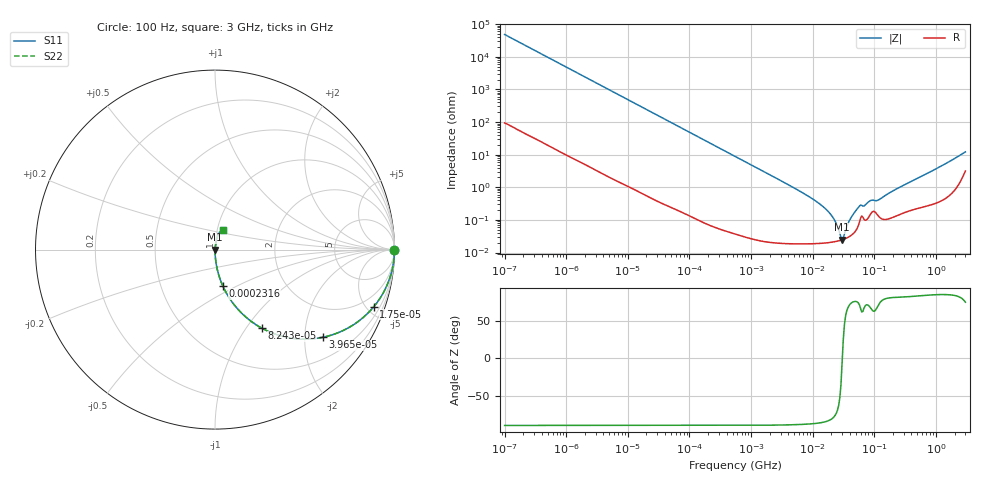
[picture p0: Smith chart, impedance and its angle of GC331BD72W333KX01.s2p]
!Murata Part Number: GC331BD72W333KX01
!These Parameters are Measured in Series Mode Connection
!Data Generated on Jun 10, 2025
!  o--ll--o
!Port1  Port2
!  o------o
!Operation Temp=25[degC], DC Bias Voltage=0[V]
!Freq. Start=100[Hz] Stop=3[GHz] 401[Steps]
# Hz S RI R 50
!Freq.(Hz) S11(Real) S11(Imag) S21(Real) S21(Imag) S12(Real) S12(Imag) S22(Real) S22(Imag)
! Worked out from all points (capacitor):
!   401 points, 100 Hz to 3 GHz, reference 50 ohm
!   read as one part in series: C = 32.9 nF near 109 Hz
!   lowest |Z| = 24.7 mohm at 29.99 MHz (marker M1)
!   series resonance near 30.23 MHz, so ESL is about 840 pH
!   S11 on the Smith chart (normalised r, x): 100 Hz: open; 17.5 kHz: 1.01, -5.56; 39.66 kHz: 1.01, -2.46; 82.43 kHz: 1.00, -1.18; 231.6 kHz: 1.00, -0.42; 3 GHz: 1.06, +0.24
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100  1 -0.00207  8.3e-06 0.00207  8.3e-06 0.00207  1 -0.00207
1788  0.9986 -0.0368  0.00143 0.0368  0.00143 0.0368  0.9986 -0.0368
6230  0.9836 -0.126  0.0164 0.126  0.0164 0.126  0.9836 -0.126
17504  0.885 -0.318  0.115 0.318  0.115 0.318  0.885 -0.318
31977  0.6985 -0.4578  0.3015 0.4578  0.3015 0.4578  0.6985 -0.4578
39655  0.6014 -0.4884  0.3986 0.4884  0.3986 0.4884  0.6014 -0.4884
82428  0.26 -0.4373  0.74 0.4373  0.74 0.4373  0.26 -0.4373
132342  0.1205 -0.3241  0.8795 0.3241  0.8795 0.3241  0.1205 -0.3241
231582  0.0432 -0.2017  0.9568 0.2017  0.9568 0.2017  0.0432 -0.2017
547723  0.00827 -0.0885  0.9917 0.0885  0.9917 0.0885  0.00827 -0.0885
9794414  0.000206 -0.00449  0.9998 0.00449  0.9998 0.00449  0.000206 -0.00449
1.950129e7  0.000208 -0.00148  0.9998 0.00148  0.9998 0.00148  0.000208 -0.00148
2.316512e7  0.000218 -0.000883  0.9998 0.000883  0.9998 0.000883  0.000218 -0.000883
2.751729e7  0.000234 -0.00031  0.9998 0.00031  0.9998 0.00031  0.000234 -0.00031
2.999103e7  0.000246 -2.54e-05  0.9998 2.54e-05  0.9998 2.54e-05  0.000246 -2.54e-05
3.268714e7  0.000261 0.000261  0.9997 -0.000261  0.9997 -0.000261  0.000261 0.000261
4.0536e7  0.000321 0.00101  0.9997 -0.00101  0.9997 -0.00101  0.000321 0.00101
5.478864e7  0.000666 0.00231  0.9993 -0.00231  0.9993 -0.00231  0.000666 0.00231
8.79653e7  0.00158 0.00363  0.9984 -0.00363  0.9984 -0.00363  0.00158 0.00363
1.188943e8  0.00127 0.00398  0.9987 -0.00398  0.9987 -0.00398  0.00127 0.00398
1.751444e8  0.00114 0.00663  0.9989 -0.00663  0.9989 -0.00663  0.00114 0.00663
3e9  0.0431 0.1091  0.9569 -0.1091  0.9569 -0.1091  0.0431 0.1091
